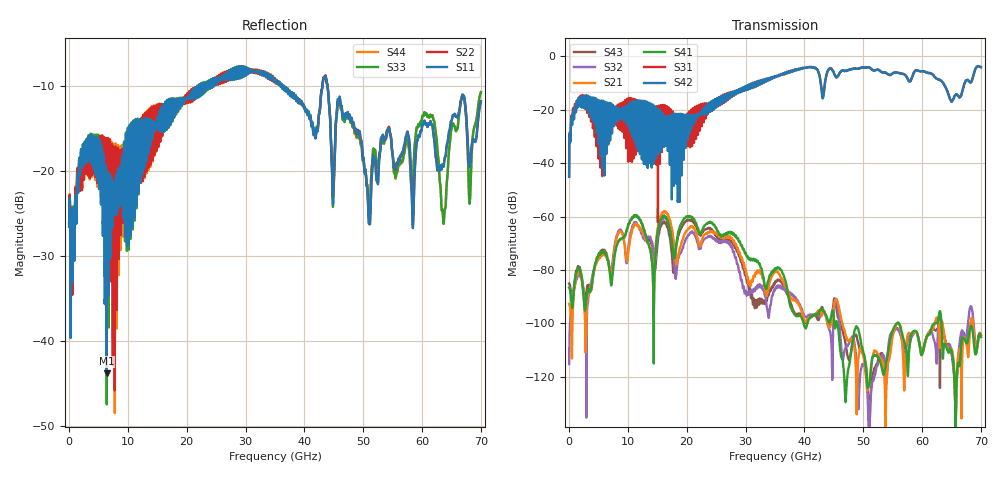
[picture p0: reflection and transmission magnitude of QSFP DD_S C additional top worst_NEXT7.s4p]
! AWR Design Environment (8415) Fri Dec 21 09:13:22 2018
! Document = 'CHANNEL TEST'
! nPorts: 4, nXvals: 7001
# HZ S DB R 50
!Freq DBS11 AngS11 DBS12 AngS12 DBS13 AngS13 DBS14 AngS14
!	DBS21 AngS21 DBS22 AngS22 DBS23 AngS23 DBS24 AngS24
!	DBS31 AngS31 DBS32 AngS32 DBS33 AngS33 DBS34 AngS34
!	DBS41 AngS41 DBS42 AngS42 DBS43 AngS43 DBS44 AngS44
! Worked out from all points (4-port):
!   7000 points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, 10 MHz to 70 GHz, reference 50 ohm
!   strongest paths, dB at 10 MHz, 17.51 GHz, 35.01 GHz, 52.51 GHz, 70 GHz:
!     S42: -45.1, -30.2, -7.6, -5.0, -4.0
!     S31: -45.1, -23.1, -7.6, -5.0, -4.0
!     S41: -86.6, -69.6, -79.7, -112.5, -105.1
!     S21: -92.7, -64.8, -80.7, -111.5, -104.3
!     S32: -115.2, -68.8, -87.5, -115.0, -104.3
!     S43: -85.0, -74.9, -84.8, -113.9, -105.1
!   lowest |S11| = -43.8 dB at 6.41 GHz (marker M1), VSWR 1.01, Z = 50.5 - j0.428 ohm
!   |S11| at or under -10 dB: start of sweep to 21.78 GHz; 36.52 GHz to 43.04 GHz (6.515 GHz wide, 16.4 % of centre); 43.91 GHz to end of sweep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
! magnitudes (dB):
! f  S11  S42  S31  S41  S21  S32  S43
! 10 MHz  -26.5  -45.1  -45.1  -86.6  -92.7  -115.2  -85.0
! 1.65 GHz  -19.9  -15.5  -15.4  -79.8  -80.9  -82.2  -79.0
! 6.41 GHz  -43.8  -20.1  -18.7  -74.8  -75.2  -75.2  -74.2
! 14.31 GHz  -14.1  -22.3  -19.9  -86.5  -87.7  -72.4  -73.5
! 16.22 GHz  -15.3  -22.4  -18.9  -59.7  -58.0  -60.2  -62.0
! 18.19 GHz  -13.2  -28.7  -24.6  -70.8  -77.4  -82.6  -71.6
! 70 GHz  -11.8  -4.0  -4.0  -105.1  -104.3  -104.3  -105.1
